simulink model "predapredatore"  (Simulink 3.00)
settings: Solver=ode45  StartTime=0.0  StopTime=25.0  RelTol=1e-6
libraries: simulink3 x1

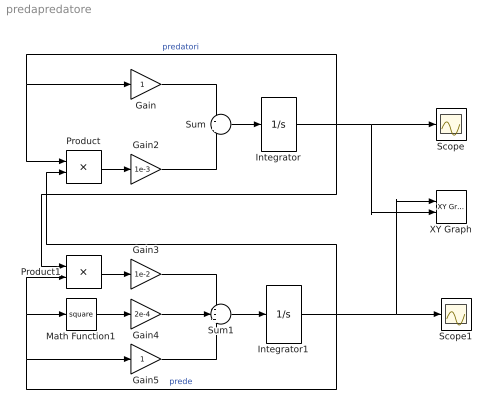
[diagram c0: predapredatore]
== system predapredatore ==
  Gain : Gain  Gain=1  SaturateOnIntegerOverflow=on
  Gain2 : Gain  Gain=1e-3  SaturateOnIntegerOverflow=on
  Gain3 : Gain  Gain=1e-2  SaturateOnIntegerOverflow=on
  Gain4 : Gain  Gain=2e-4  SaturateOnIntegerOverflow=on
  Gain5 : Gain  Gain=1  SaturateOnIntegerOverflow=on
  Integrator : Integrator  ExternalReset=none  InitialConditionSource=internal  InitialCondition=200  LimitOutput=on  UpperSaturationLimit=inf  LowerSaturationLimit=-inf  ShowSaturationPort=off  ShowStatePort=off  AbsoluteTolerance=auto
  Integrator1 : Integrator  ExternalReset=none  InitialConditionSource=internal  InitialCondition=2000  LimitOutput=on  UpperSaturationLimit=inf  LowerSaturationLimit=-inf  ShowSaturationPort=off  ShowStatePort=off  AbsoluteTolerance=auto
  Math Function1 : Math  Operator=square  OutputSignalType=auto
  Product : Product  Inputs=2  SaturateOnIntegerOverflow=on
  Product1 : Product  Inputs=2  SaturateOnIntegerOverflow=on
  Scope : Scope
  Scope1 : Scope
  Sum : Sum  Inputs=-+  SaturateOnIntegerOverflow=on
  Sum1 : Sum  Inputs=--+  SaturateOnIntegerOverflow=on
  XY Graph : simulink3/Sinks/XY Graph  xmin=0  xmax=5000  ymin=0  ymax=500  st=-1
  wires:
  Product/1 -> Gain2/1
  Gain/1 -> Sum/1
  Sum/1 -> Integrator/1
  Math Function1/1 -> Gain4/1
  Gain3/1 -> Sum1/1
  Gain4/1 -> Sum1/2
  Sum1/1 -> Integrator1/1
  Integrator/1 -> Gain/1, Product/1, Product1/1, Scope/1, XY Graph/2  "predatori"
  Product1/1 -> Gain3/1
  Integrator1/1 -> Gain5/1, Math Function1/1, Product1/2, Product/2, Scope1/1, XY Graph/1  "prede"
  Gain5/1 -> Sum1/3
  Gain2/1 -> Sum/2
